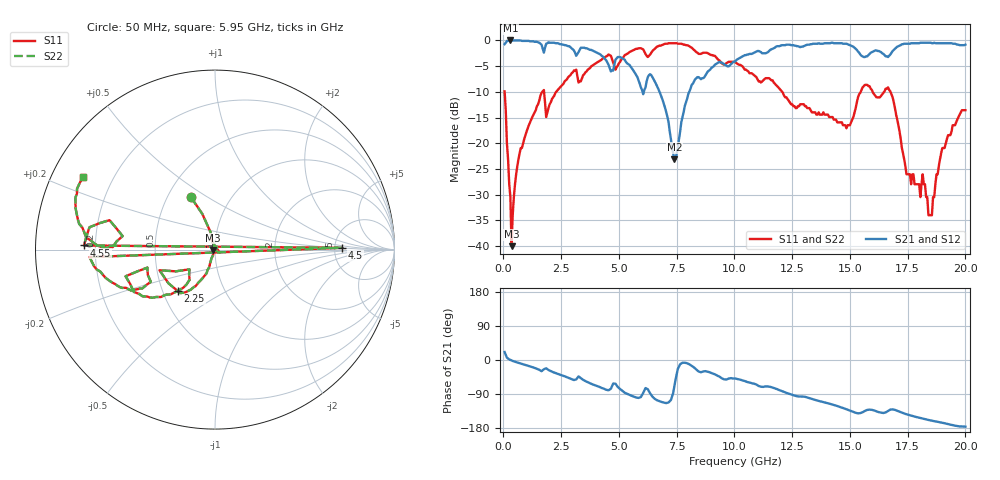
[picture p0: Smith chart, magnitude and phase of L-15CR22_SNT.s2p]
#	mhz	s	ma	r	50
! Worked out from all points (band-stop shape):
!   400 points, 50 MHz to 20 GHz, reference 50 ohm
!   highest |S21| = 0.00 dB at 300 MHz (marker M1); lowest = -23.1 dB at 7.4 GHz (marker M2)
!   |S21| within 3 dB of the highest: start of sweep to 4.26 GHz; 10.39 GHz to 15.51 GHz (5.12 GHz wide, 39.5 % of centre)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
!   lowest |S11| = -40.0 dB at 350 MHz (marker M3), VSWR 1.02, Z = 49 - j0.164 ohm
!   |S11| at or under -10 dB: 51.41 MHz to 1.681 GHz (1.63 GHz wide, 188 % of centre); 12.07 GHz to 15.47 GHz (3.397 GHz wide, 24.7 % of centre); 16.76 GHz to end of sweep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
!   |S22| runs from -40.0 to -0.5 dB; largest |S21 - S12| = 0
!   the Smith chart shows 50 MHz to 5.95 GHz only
!   S11 on the Smith chart (normalised r, x): 50 MHz: 0.66, +0.43; 2.25 GHz: 0.60, -0.31; 4.5 GHz: 5.89, +0.24; 4.55 GHz: 0.16, +0.02; 5.95 GHz: 0.09, +0.26
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50  0.32 114.6  0.92 21.0  0.92 21.0  0.32 114.6
300  0.03 -30.9  1 0.2  1 0.2  0.03 -30.9
350  0.01 -170.4  1 -1.3  1 -1.3  0.01 -170.4
750  0.09 -109.2  1 -9.4  1 -9.4  0.09 -109.2
2250  0.31 -131.6  0.94 -34.1  0.94 -34.1  0.31 -131.6
3400  0.43 -152.7  0.85 -50.2  0.85 -50.2  0.43 -152.7
4450  0.7 -176.6  0.64 -78.6  0.64 -78.6  0.7 -176.6
4500  0.71 0.8  0.61 -79.2  0.61 -79.2  0.71 0.8
4550  0.73 178.2  0.58 -79.9  0.58 -79.9  0.73 178.2
5950  0.84 151.0  0.35 -97.8  0.35 -97.8  0.84 151.0
6700  0.88 146.8  0.34 -107.4  0.34 -107.4  0.88 146.8
7400  0.94 121.7  0.07 -69.4  0.07 -69.4  0.94 121.7
8300  0.79 82.4  0.42 -22.5  0.42 -22.5  0.79 82.4
10050  0.61 60.8  0.63 -48.9  0.63 -48.9  0.61 60.8
13350  0.2 22.1  0.92 -102.5  0.92 -102.5  0.2 22.1
15150  0.18 34.5  0.87 -137.1  0.87 -137.1  0.18 34.5
16700  0.33 20.4  0.71 -132.7  0.71 -132.7  0.33 20.4
17450  0.05 28.6  0.93 -143.2  0.93 -143.2  0.05 28.6
18150  0.05 111.7  0.95 -154.4  0.95 -154.4  0.05 111.7
18400  0.02 87.8  0.95 -158.2  0.95 -158.2  0.02 87.8
19000  0.09 -49.4  0.94 -165.7  0.94 -165.7  0.09 -49.4
20000  0.21 -59.2  0.91 -176.0  0.91 -176.0  0.21 -59.2
